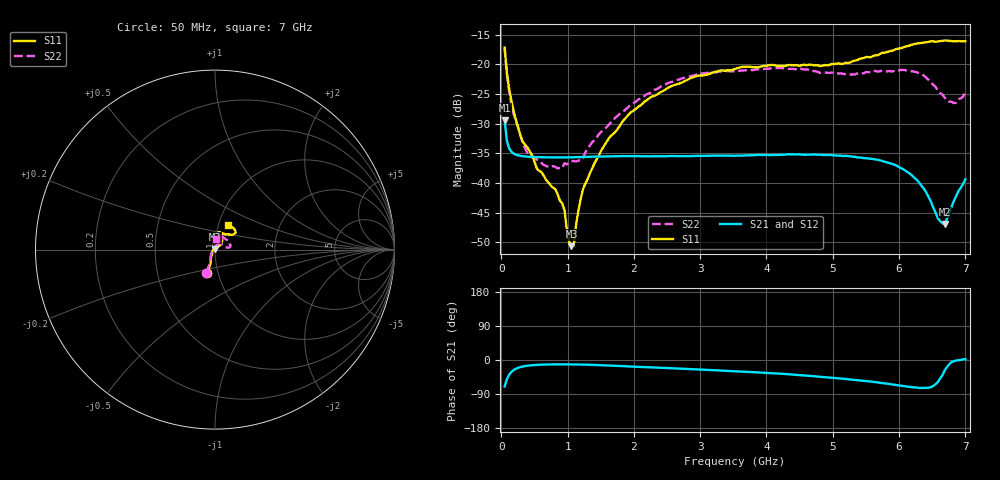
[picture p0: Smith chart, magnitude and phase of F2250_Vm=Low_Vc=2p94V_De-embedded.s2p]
! Integrated Device Technology
! Corporate Headquarters
! 6024 Silver Creek Valley Road
! San Jose, CA 95138  USA
! Phone:  1-408-284-8200
! Toll Free:  1-800-223-1366
! Webpage:  http://www.idt.com/
! Timing and RF Division
! 515 Groton Road, Suite 102
! Westford, MA 01886-6024
! Device:  F2250
! Description: Voltage Variable RF Attenuator
! Frequency:  50.0 -  6000.00 MHz
! Package:  3x3 mm Thin QFN Plastic Package: 16 pin
! Ports:  2 RF, 3 DC
!  Pin  1  = GND
!  Pin  2  = NC
!  Pin  3  = RF1  = Port 1
!  Pin  4  = NC
!  Pin  5  = GND
!  Pin  6  = GND
!  Pin  7  = GND
!  Pin  8  = GND
!  Pin  9  = NC
!  Pin 10  = RF2  = Port 2
!  Pin 11  = NC
!  Pin 12  = GND
!  Pin 13  = GND
!  Pin 14  = VCNTRL
!  Pin 15  = VDD
!  Pin 16  = VMODE
! Vcntrl:  2.940 Volts
! Vmode:  +0.000 Volts
! Vdd:  +3.30  Volts
! Current:  1.177 mA
! Data:  The device was measured on a the F2250 evaluation board which has
!  individual transmission lines to the RF pins.  Data was collected
!  using a calibrated network analyzer.  The evaluation board was
!  de-embedded using a TRL calibration technique.
!  The reference plane is the edge of the package pin.
! Misc:  SN 10
!  Action Tracker AT0258
! Date Measured:  2014-11-26
! Date:  2015-10-15  MJV
! Note:
!  Integrated Device Technology supplies this data as a sample of measured
!  data at the package pin for this product.  Your particular data for this
!  product may vary.
!  Data was taken at 25 degrees C.
!  Integrated Device Technology reserves the right to change this data at anytime.
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# GHz S dB R 50
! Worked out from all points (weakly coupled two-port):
!   201 points, 50 MHz to 7 GHz, reference 50 ohm
!   highest |S21| = -29.41 dB at 50 MHz (marker M1); lowest = -46.9 dB at 6.687 GHz (marker M2)
!   lowest |S11| = -50.6 dB at 1.058 GHz (marker M3), VSWR 1.01, Z = 49.8 + j0.243 ohm
!   |S11| at or under -10 dB: start of sweep to end of sweep
!   |S22| runs from -37.5 to -17.3 dB; largest |S21 - S12| = 6.2e-05
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0.05  -17.18 -108.6  -29.41 -69.8  -29.41 -69.8  -17.28 -111.0
0.08475  -21.45 -107.5  -32.92 -50.4  -32.92 -50.4  -21.75 -110.2
0.15425  -26.23 -116.6  -34.76 -31.1  -34.75 -31.1  -26.82 -122.5
0.29325  -32.21 -127.9  -35.43 -18.5  -35.43 -18.5  -32.10 -137.5
0.3975  -34.09 -141.9  -35.56 -15.0  -35.56 -15.0  -35.04 -160.6
0.5365  -37.55 -155.6  -35.64 -12.8  -35.64 -12.8  -36.04 178.0
0.91875  -43.44 157.7  -35.69 -11.5  -35.68 -11.5  -37.53 133.5
0.9535  -44.57 170.1  -35.68 -11.5  -35.68 -11.5  -36.66 131.2
1.023  -49.89 143.1  -35.68 -11.6  -35.68 -11.6  -36.62 116.0
1.05775  -50.63 124.0  -35.67 -11.7  -35.67 -11.6  -36.29 110.8
1.0925  -50.46 89.5  -35.66 -11.7  -35.66 -11.7  -36.29 106.3
1.162  -44.71 56.9  -35.64 -11.9  -35.64 -11.9  -36.22 95.6
1.2315  -41.08 44.4  -35.61 -12.1  -35.61 -12.1  -35.78 85.8
1.6485  -32.11 42.0  -35.52 -14.7  -35.52 -14.6  -29.87 64.6
2.37825  -24.86 47.3  -35.47 -20.3  -35.48 -20.3  -23.98 56.8
3.525  -20.79 72.5  -35.40 -29.5  -35.40 -29.5  -21.19 74.7
4.7065  -20.17 72.3  -35.19 -42.6  -35.19 -42.6  -21.14 72.2
5.85325  -17.82 40.4  -36.64 -63.4  -36.63 -63.5  -21.14 23.1
6.27025  -16.51 40.0  -39.49 -72.8  -39.50 -72.9  -21.37 9.7
6.68725  -15.99 48.7  -46.90 -27.7  -46.89 -27.5  -25.62 28.7
6.861  -16.14 55.1  -42.19 -1.3  -42.15 -1.3  -26.45 57.9
7  -16.13 63.2  -39.38 1.9  -39.34 1.7  -24.63 83.1
